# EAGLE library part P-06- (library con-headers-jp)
HEADER PLUG PINS
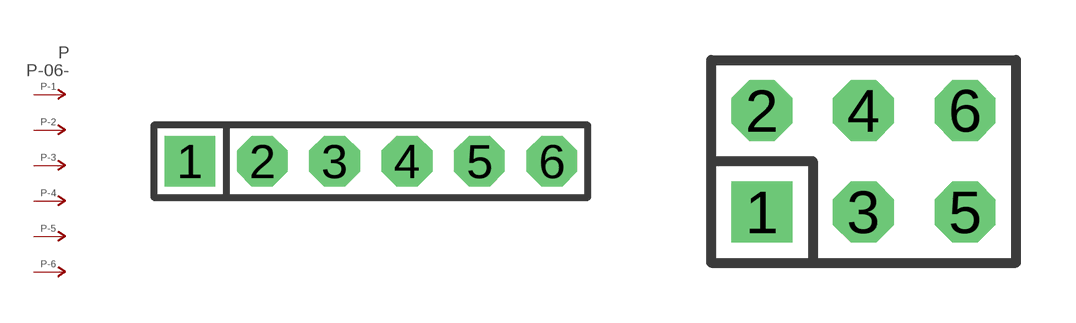
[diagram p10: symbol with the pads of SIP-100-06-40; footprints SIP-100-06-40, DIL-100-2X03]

Designator prefix P; gates -2=P-N -3=P-N -4=P-N -5=P-N -6=P-N -1=P-NV

## P-06-SIP-100-40  [SIP-100-06-40]
1  -1:P  pas
2  -2:P  pas
3  -3:P  pas
4  -4:P  pas
5  -5:P  pas
6  -6:P  pas

## P-06-100-2X03  [DIL-100-2X03]
Pads as for SIP-100-06-40

## P-06-100-2X03_M  [DIL-100-2X03_M]
Pads as for SIP-100-06-40

## P-06-2MM-2X03  [DIL-2MM-2X03]
Pads as for SIP-100-06-40

## P-06-2MM-2X03_M  [DIL-2MM-2X03_M]
Pads as for SIP-100-06-40

## P-06-SIP-100-32  [SIP-100-06-32]
Pads as for SIP-100-06-40

## P-06-SIP-100-40Y  [SIP-100-06-40Y]
Pads as for SIP-100-06-40

## P-06-SIP-100-32Y  [SIP-100-06-32Y]
Pads as for SIP-100-06-40

## P-06-LCW-106-XX-X-S  [LCW-106-XX-X-S]
Pads as for SIP-100-06-40

## P-06-LCW-106-XX-X-S-RE  [LCW-106-XX-X-S-RE]
Pads as for SIP-100-06-40

## Footprint SIP-100-06-40 (pad centres in mm)
SIP Header - 0.1", 40 mil drill
drill 1.016 pad 1.778 square: 1 -6.35,0
drill 1.016 pad 1.778 octagon: 2 -3.81,0; 3 -1.27,0; 4 1.27,0; 5 3.81,0; 6 6.35,0

## Footprint DIL-100-2X03 (pad centres in mm)
PIN HEADER - 0.1"
drill 1.016 square: 1 -2.54,-1.27
drill 1.016 octagon: 2 -2.54,1.27; 3 0,-1.27; 4 0,1.27; 5 2.54,-1.27; 6 2.54,1.27

## Footprint DIL-100-2X03_M (pad centres in mm)
PIN HEADER - MIRRORED 0.1"
drill 1.016 square: 1 -2.54,1.27
drill 1.016 octagon: 2 -2.54,-1.27; 3 0,1.27; 4 0,-1.27; 5 2.54,1.27; 6 2.54,-1.27

## Footprint DIL-2MM-2X03 (pad centres in mm)
PIN HEADER - 2MM"
drill 0.711 square: 1 -2,-1
drill 0.711: 2 -2,1; 3 0,-1; 4 0,1; 5 2,-1; 6 2,1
